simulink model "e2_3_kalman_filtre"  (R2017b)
settings: Solver=FixedStepAuto  StartTime=0.0  StopTime=30  FixedStep=fixed_step_size  RelTol=1e-3
StopFcn:
  | if AUTOLAND
  | %1_2
  | land1 = rospublisher('/tello1/land','std_msgs/Empty');
  | msg=rosmessage(land1);
  | send(land1,msg);
  | land2 = rospublisher('/tello2/land','std_msgs/Empty');
  | msg=rosmessage(land2);
  | send(land2,msg);
  | %3_4
  | land3 = rospublisher('/tello3/land','std_msgs/Empty');
  | msg=rosmessage(land3);
  | send(land3,msg);
  | land4 = rospublisher('/tello4/land','std_msgs/Empty');
  | msg=rosmessage(land4);
  | send(land4,msg);
  | %5_6
  | land5 = rospublisher('/tello5/land','std_msgs/Empty');
  | msg=rosmessage(land5);
  | send(land5,msg);
  | land6= rospublisher('/tello6/land','std_msgs/Empty');
  | msg=rosmessage(land6);
  | send(land6,msg);
  | %7_8
  | land7 = rospublisher('/tello7/land','std_msgs/Empty');
  | msg=rosmessage(land7);
  | send(land7,msg);
  | land8 = rospublisher('/tello8/land','std_msgs/Empty');
  | msg=rosmessage(land8);
  | send(land8,msg);
  | end
  | 
  | generate_cifer_datapack
  | 
  | if TELLO_PLOT
  | tello8_plot
  | end
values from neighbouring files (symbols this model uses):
  a = XMAX    (= 0.8)    [start_tello.m]
  b = YMAX    (= 1.2)    [start_tello.m]
  battery_threshold = 15    [start_tello.m]
  bb = (ZMIN*YMAX - ZMAX*YMIN)/(YMAX - YMIN)    (= -1.05)    [start_tello.m]
  fcnCmdMag = 1    [start.m]
  fcnNumber = 4    [start.m]
  fcnSinFreq = 50.0    (= 50)    [start.m]
  high_time = 5    [start.m]
  k = (ZMAX - ZMIN)/(YMAX - YMIN)    (= 0.458333333333)    [start_tello.m]
  omega = 1.0    (= 1)    [start.m]    (also in start_tello.m = 0.3)
  PARAM_C1 = 4.0    (= 4)    [start.m]
  PARAM_C2 = 0.0187    [start.m]
  PARAM_isNoiseOn = false    [start.m]
  PARAM_T_rec = ceil(5*2*pi/PARAM_w_min)    [start.m]
  PARAM_time_end = PARAM_time_start + 20    (= 23)    [start.m]
  PARAM_time_start = 3    [start.m]
  PARAM_w_max = 12    [start.m]
  PARAM_w_min = 0.5    [start.m]
  R = 1.0    (= 1)    [start.m]    (also in start_tello.m)
  sim_end_time = 15*act_end + 4    (= 475.238898038)    [start_tello.m]
  step_period = zero1_time+high_time+zero2_time+low_time    (= 18)    [start.m]
  tb2 = tb    (= 2.7)    [start_tello.m]
  tb3 = tb*2    (= 5.4)    [start_tello.m]
  tb4 = tb*3    (= 8.1)    [start_tello.m]
  tb5 = tb*4    (= 10.8)    [start_tello.m]
  tb6 = tb*5    (= 13.5)    [start_tello.m]
  tb7 = tb*6    (= 16.2)    [start_tello.m]
  tb8 = tb*7    (= 18.9)    [start_tello.m]
  TELLO1_NUM = uint8(1)    [start_tello.m]
  TELLO2_NUM = uint8(2)    [start_tello.m]
  TELLO3_NUM = uint8(3)    [start_tello.m]
  TELLO4_NUM = uint8(4)    [start_tello.m]
  TELLO5_NUM = uint8(5)    [start_tello.m]
  TELLO6_NUM = uint8(6)    [start_tello.m]
  TELLO7_NUM = uint8(7)    [start_tello.m]
  TELLO8_NUM = uint8(8)    [start_tello.m]
  UAV_NUM = 0    [start_tello.m]
  w1 = 0.4    [start_tello.m]
  w2 = 0.2    [start_tello.m]
  z_d_for_land = -0.2    [start_tello.m]
  zero1_time = 3    [start.m]
  zero2_time = 5    [start.m]
  zero3_time = 5    [start.m]
undefined symbols (not defined in the file or in its folder): DiscIntNeverNeededParam, sigbuilder_block
libraries: simulink x45, etargetslib x24, dspnetwork x24, sharedtransform x8, aerolibanimutils x1
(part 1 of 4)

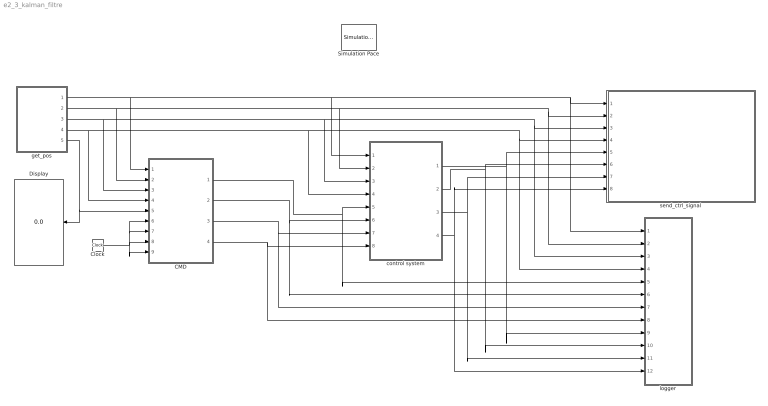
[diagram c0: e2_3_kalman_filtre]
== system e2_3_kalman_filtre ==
  CMD : Subsystem
  Clock : Clock
  Display : Display
  Simulation Pace : aerolibanimutils/Simulation Pace  SimulationPace=1  SleepMode=MATLAB Thread  OutputPaceError=off  SampleTime=-1
  control system : Subsystem
  get_pos : Subsystem
  logger : Subsystem  Commented=on
  send_ctrl_signal : Subsystem
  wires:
  control system/1(output1_2) -> logger/9(u1_2), send_ctrl_signal/5(control1_2)
  CMD/1(state_d1_2) -> logger/5(state_d1_2), control system/5(state_d1_2)
  CMD/2(state_d3_4) -> logger/6(state_d3_4), control system/6(state_d3_4)
  CMD/3(state_d5_6) -> logger/7(state_d5_6), control system/7(state_d5_6)
  CMD/4(state_d7_8) -> control system/8(state_d7_8), logger/8(state_d7_8)
  control system/2(output3_4) -> logger/10(u3_4), send_ctrl_signal/6(control3_4)
  control system/3(output5_6) -> logger/11(u5_6), send_ctrl_signal/7(control5_6)
  control system/4(output7_8) -> logger/12(u7_8), send_ctrl_signal/8(control7_8)
  get_pos/1(tello1_2) -> CMD/1(telo_state1_2), send_ctrl_signal/1(state1_2), logger/1(state1_2), control system/1(state1_2)
  get_pos/2(tello3_4) -> CMD/2(telo_state3_4), logger/2(state3_4), send_ctrl_signal/2(state3_4), control system/2(state3_4)
  get_pos/3(tello5_6) -> CMD/3(telo_state5_6), logger/3(state5_6), send_ctrl_signal/3(state5_6), control system/3(state5_6)
  get_pos/4(tello7_8) -> CMD/4(telo_state7_8), logger/4(state7_8), send_ctrl_signal/4(state7_8), control system/4(state7_8)
  Clock/1 -> CMD/6(clock1_2), CMD/7(clock3_4), CMD/8(clock5_6), CMD/9(clock7_8)
  get_pos/5(tello_bat) -> Display/1, CMD/5(tello_bat)

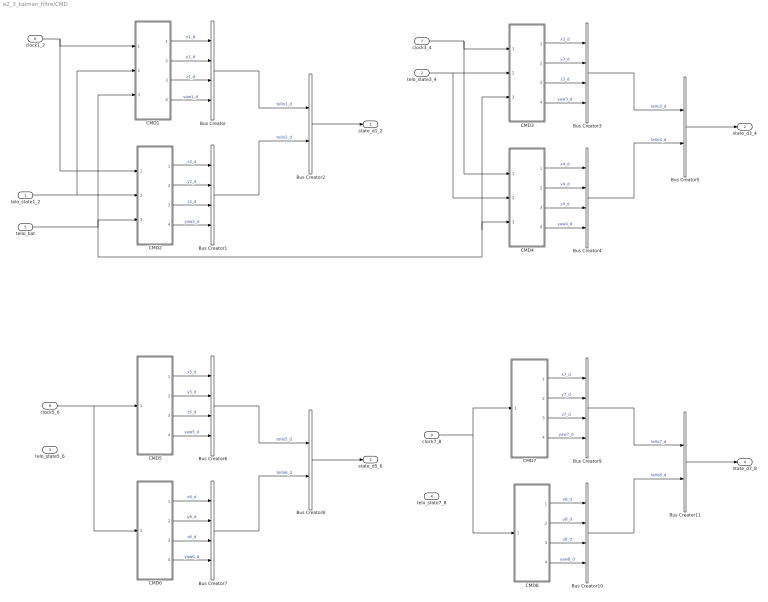
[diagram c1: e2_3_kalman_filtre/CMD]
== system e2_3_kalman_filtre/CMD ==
  telo_state1_2 : Inport
  telo_state3_4 : Inport  Port=2
  telo_state5_6 : Inport  Port=3
  telo_state7_8 : Inport  Port=4
  tello_bat : Inport  Port=5
  clock1_2 : Inport  Port=6
  clock3_4 : Inport  Port=7
  clock5_6 : Inport  Port=8
  clock7_8 : Inport  Port=9
  Bus Creator{,1,3..4,6..7,9..10} (8 alike) : BusCreator  Inputs=4
  Bus Creator{2,5,8,11} (4 alike) : BusCreator  Inputs=2
  CMD1 : Subsystem
  CMD2 : Subsystem
  CMD3 : Subsystem
  CMD4 : Subsystem
  CMD5 : Subsystem
  CMD6 : Subsystem
  CMD7 : Subsystem
  CMD8 : Subsystem
  state_d1_2 : Outport
  state_d3_4 : Outport  Port=2
  state_d5_6 : Outport  Port=3
  state_d7_8 : Outport  Port=4
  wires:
  CMD1/1(x_d) -> Bus Creator/1  "x1_d"
  CMD1/2(y_d) -> Bus Creator/2  "y1_d"
  CMD1/3(z_d) -> Bus Creator/3  "z1_d"
  CMD1/4(yaw_d) -> Bus Creator/4  "yaw1_d"
  CMD2/1(x_d) -> Bus Creator1/1  "x2_d"
  CMD2/2(y_d) -> Bus Creator1/2  "y2_d"
  CMD2/3(z_d) -> Bus Creator1/3  "z2_d"
  CMD2/4(yaw_d) -> Bus Creator1/4  "yaw2_d"
  Bus Creator/1 -> Bus Creator2/1  "tello1_d"
  Bus Creator1/1 -> Bus Creator2/2  "tello2_d"
  Bus Creator2/1 -> state_d1_2/1
  Bus Creator3/1 -> Bus Creator5/1  "tello3_d"
  Bus Creator4/1 -> Bus Creator5/2  "tello4_d"
  CMD3/2(y_d) -> Bus Creator3/2  "y3_d"
  CMD3/3(z_d) -> Bus Creator3/3  "z3_d"
  CMD3/4(yaw_d) -> Bus Creator3/4  "yaw3_d"
  Bus Creator5/1 -> state_d3_4/1
  CMD4/1(x_d) -> Bus Creator4/1  "x4_d"
  CMD3/1(x_d) -> Bus Creator3/1  "x3_d"
  CMD4/2(y_d) -> Bus Creator4/2  "y4_d"
  CMD4/4(yaw_d) -> Bus Creator4/4  "yaw4_d"
  CMD4/3(z_d) -> Bus Creator4/3  "z4_d"
  CMD5/2(y_d) -> Bus Creator6/2  "y5_d"
  Bus Creator11/1 -> state_d7_8/1
  CMD7/3(z_d) -> Bus Creator9/3  "z7_d"
  Bus Creator6/1 -> Bus Creator8/1  "tello5_d"
  CMD8/3(z_d) -> Bus Creator10/3  "z8_d"
  CMD8/4(yaw_d) -> Bus Creator10/4  "yaw8_d"
  CMD5/3(z_d) -> Bus Creator6/3  "z5_d"
  CMD7/4(yaw_d) -> Bus Creator9/4  "yaw7_d"
  CMD5/4(yaw_d) -> Bus Creator6/4  "yaw5_d"
  CMD7/2(y_d) -> Bus Creator9/2  "y7_d"
  Bus Creator7/1 -> Bus Creator8/2  "tello6_d"
  CMD8/1(x_d) -> Bus Creator10/1  "x8_d"
  Bus Creator9/1 -> Bus Creator11/1  "tello7_d"
  Bus Creator10/1 -> Bus Creator11/2  "tello8_d"
  clock1_2/1 -> CMD2/1("clock "), CMD1/1("clock ")
  CMD6/2(y_d) -> Bus Creator7/2  "y6_d"
  CMD6/4(yaw_d) -> Bus Creator7/4  "yaw6_d"
  CMD6/1(x_d) -> Bus Creator7/1  "x6_d"
  CMD7/1(x_d) -> Bus Creator9/1  "x7_d"
  CMD5/1(x_d) -> Bus Creator6/1  "x5_d"
  Bus Creator8/1 -> state_d5_6/1
  CMD8/2(y_d) -> Bus Creator10/2  "y8_d"
  CMD6/3(z_d) -> Bus Creator7/3  "z6_d"
  clock5_6/1 -> CMD6/1("clock "), CMD5/1("clock ")
  clock7_8/1 -> CMD7/1("clock "), CMD8/1("clock ")
  clock3_4/1 -> CMD4/1("clock "), CMD3/1("clock ")
  telo_state1_2/1 -> CMD1/2(tello_states), CMD2/2(tello_states)
  tello_bat/1 -> CMD1/3(tello_bat), CMD3/3(tello_bat), CMD4/3(tello_bat), CMD2/3(tello_bat)
  telo_state3_4/1 -> CMD4/2(tello_states), CMD3/2(tello_states)

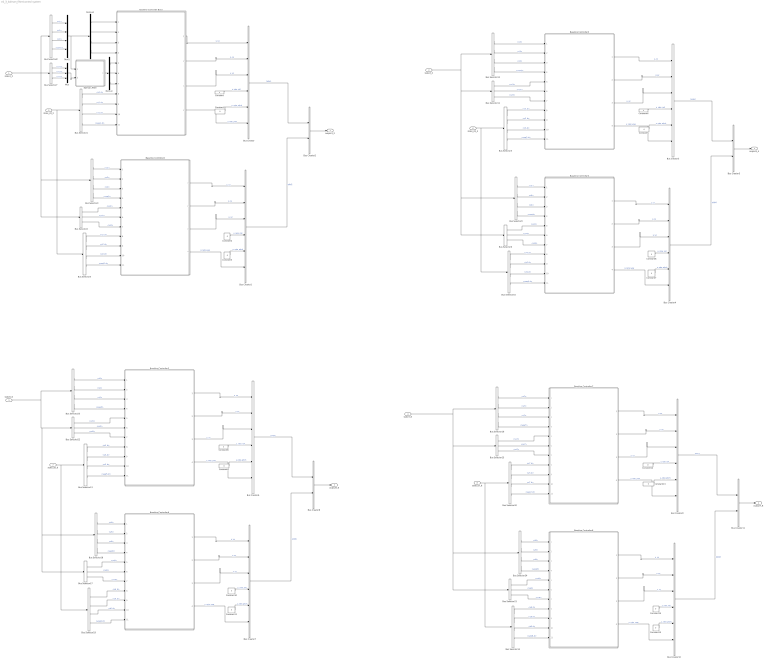
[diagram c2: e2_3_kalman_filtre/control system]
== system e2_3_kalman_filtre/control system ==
  state1_2 : Inport
  state3_4 : Inport  Port=2
  state5_6 : Inport  Port=3
  state7_8 : Inport  Port=4
  state_d1_2 : Inport  Port=5
  state_d3_4 : Inport  Port=6
  state_d5_6 : Inport  Port=7
  state_d7_8 : Inport  Port=8
  Baseline Controller Basic : Subsystem  AncestorBlock=ARBlocks/Baseline Controller
  Baseline Controller2 : Subsystem  AncestorBlock=ARBlocks/Baseline Controller
  Baseline Controller3 : Subsystem  AncestorBlock=ARBlocks/Baseline Controller
  Baseline Controller4 : Subsystem  AncestorBlock=ARBlocks/Baseline Controller
  Baseline Controller5 : Subsystem  AncestorBlock=ARBlocks/Baseline Controller
  Baseline Controller6 : Subsystem  AncestorBlock=ARBlocks/Baseline Controller
  Baseline Controller7 : Subsystem  AncestorBlock=ARBlocks/Baseline Controller
  Baseline Controller8 : Subsystem  AncestorBlock=ARBlocks/Baseline Controller
  Bus Creator{,1,3..4,6..7,9..10} (8 alike) : BusCreator  Inputs=6
  Bus Creator{2,5,8,11} (4 alike) : BusCreator  Inputs=2
  Bus Selector1 : BusSelector  OutputSignals=tello1_d.x1_d,tello1_d.y1_d,tello1_d.z1_d,tello1_d.yaw1_d
  Bus Selector10 : BusSelector  OutputSignals=tello4_d.x4_d,tello4_d.y4_d,tello4_d.z4_d,tello4_d.yaw4_d
  Bus Selector11 : BusSelector  OutputSignals=tello3_states.vx3,tello3_states.vy3,tello3_states.vz3
  Bus Selector12 : BusSelector  OutputSignals=tello3_states.x3,tello3_states.y3,tello3_states.z3,tello3_states.yaw3
  Bus Selector13 : BusSelector  OutputSignals=tello5_d.x5_d,tello5_d.y5_d,tello5_d.z5_d,tello5_d.yaw5_d
  Bus Selector14 : BusSelector  OutputSignals=tello8_d.x8_d,tello8_d.y8_d,tello8_d.z8_d,tello8_d.yaw8_d
  Bus Selector15 : BusSelector  OutputSignals=tello7_states.vx7,tello7_states.vy7,tello7_states.vz7
  Bus Selector16 : BusSelector  OutputSignals=tello7_states.x7,tello7_states.y7,tello7_states.z7,tello7_states.yaw7
  Bus Selector17 : BusSelector  OutputSignals=tello6_states.vx6,tello6_states.vy6,tello6_states.vz6
  Bus Selector18 : BusSelector  OutputSignals=tello6_states.x6,tello6_states.y6,tello6_states.z6,tello6_states.yaw6
  Bus Selector19 : BusSelector  OutputSignals=tello6_d.x6_d,tello6_d.y6_d,tello6_d.z6_d,tello6_d.yaw6_d
  Bus Selector2 : BusSelector  OutputSignals=tello2_states.vx2,tello2_states.vy2,tello2_states.vz2
  Bus Selector20 : BusSelector  OutputSignals=tello7_d.x7_d,tello7_d.y7_d,tello7_d.z7_d,tello7_d.yaw7_d
  Bus Selector21 : BusSelector  OutputSignals=tello8_states.vx8,tello8_states.vy8,tello8_states.vz8
  Bus Selector22 : BusSelector  OutputSignals=tello5_states.vx5,tello5_states.vy5,tello5_states.vz5
  Bus Selector23 : BusSelector  OutputSignals=tello5_states.x5,tello5_states.y5,tello5_states.z5,tello5_states.yaw5
  Bus Selector24 : BusSelector  OutputSignals=tello8_states.x8,tello8_states.y8,tello8_states.z8,tello8_states.yaw8
  Bus Selector3 : BusSelector  OutputSignals=tello2_states.x2,tello2_states.y2,tello2_states.z2,tello2_states.yaw2
  Bus Selector4 : BusSelector  OutputSignals=tello2_d.x2_d,tello2_d.y2_d,tello2_d.z2_d,tello2_d.yaw2_d
  Bus Selector5 : BusSelector  OutputSignals=tello3_d.x3_d,tello3_d.y3_d,tello3_d.z3_d,tello3_d.yaw3_d
  Bus Selector6 : BusSelector  OutputSignals=tello4_states.vx4,tello4_states.vy4,tello4_states.vz4
  Bus Selector7 : BusSelector  OutputSignals=tello1_states.vx1,tello1_states.vy1,tello1_states.vz1
  Bus Selector8 : BusSelector  OutputSignals=tello1_states.x1,tello1_states.y1,tello1_states.z1,tello1_states.yaw1
  Bus Selector9 : BusSelector  OutputSignals=tello4_states.x4,tello4_states.y4,tello4_states.z4,tello4_states.yaw4
  Constant{,1..15} (16 alike) : Constant  Value=0
  Demux : Demux  Outputs=3
  Demux1 : Demux
  Kalman_Filtre : Subsystem
  Mux : Mux  Inputs=3
  Mux1 : Mux
  output1_2 : Outport
  output3_4 : Outport  Port=2
  output5_6 : Outport  Port=3
  output7_8 : Outport  Port=4
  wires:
  Bus Selector1/2 -> Baseline Controller Basic/9(y_d)  "<y1_d>"
  Bus Selector8/3 -> Mux1/3  "<z1>"
  Bus Selector1/3 -> Baseline Controller Basic/10(Z_d)  "<z1_d>"
  Bus Selector8/4 -> Mux1/4  "<yaw1>"
  Bus Selector2/2 -> Baseline Controller2/6(V_y)  "<vy2>"
  Bus Selector3/4 -> Baseline Controller2/4(Yaw_e)  "<yaw2>"
  Bus Selector3/2 -> Baseline Controller2/2(Y_e)  "<y2>"
  Bus Selector1/1 -> Baseline Controller Basic/8(x_d)  "<x1_d>"
  Bus Selector7/1 -> Mux/1  "<vx1>"
  Bus Selector3/1 -> Baseline Controller2/1(X_e)  "<x2>"
  Bus Selector2/3 -> Baseline Controller2/7("V_z ")  "<vz2>"
  Bus Selector7/2 -> Mux/2  "<vy1>"
  Bus Selector2/1 -> Baseline Controller2/5(" V_x")  "<vx2>"
  Bus Selector8/1 -> Mux1/1  "<x1>"
  Bus Selector3/3 -> Baseline Controller2/3(" Z_e ")  "<z2>"
  Bus Selector1/4 -> Baseline Controller Basic/11(Yaw_d)  "<yaw1_d>"
  Bus Selector8/2 -> Mux1/2  "<y1>"
  Bus Selector7/3 -> Mux/3  "<vz1>"
  Baseline Controller Basic/1(ux) -> Bus Creator/1  "u_vx"
  Baseline Controller Basic/2(uy) -> Bus Creator/2  "u_vy"
  Baseline Controller Basic/3(Z_velocity_d. [-1,1]) -> Bus Creator/3  "u_vz"
  Baseline Controller Basic/4(yaw_rate_d [-1,1]) -> Bus Creator/6  "u_rate_yaw"
  Constant/1 -> Bus Creator/4  "u_rate_roll"
  Constant1/1 -> Bus Creator/5  "u_rate_pitch"
  Baseline Controller2/4(yaw_rate_d [-1,1]) -> Bus Creator1/6  "u_rate_yaw"
  Baseline Controller2/1(ux) -> Bus Creator1/1  "u_vx"
  Constant2/1 -> Bus Creator1/4  "u_rate_roll"
  Baseline Controller2/2(uy) -> Bus Creator1/2  "u_vy"
  Baseline Controller2/3(Z_velocity_d. [-1,1]) -> Bus Creator1/3  "u_vz"
  Constant3/1 -> Bus Creator1/5  "u_rate_pitch"
  Bus Creator/1 -> Bus Creator2/1  "tello1"
  Bus Creator1/1 -> Bus Creator2/2  "tello2"
  Bus Creator2/1 -> output1_2/1
  state_d1_2/1 -> Bus Selector4/1, Bus Selector1/1
  Bus Selector4/1 -> Baseline Controller2/8(x_d)  "<x2_d>"
  Bus Selector4/3 -> Baseline Controller2/10(Z_d)  "<z2_d>"
  Bus Selector4/2 -> Baseline Controller2/9(y_d)  "<y2_d>"
  Bus Selector4/4 -> Baseline Controller2/11(Yaw_d)  "<yaw2_d>"
  Bus Selector6/3 -> Baseline Controller4/7("V_z ")  "<vz4>"
  Bus Selector6/1 -> Baseline Controller4/5(" V_x")  "<vx4>"
  Bus Selector12/4 -> Baseline Controller3/4(Yaw_e)  "<yaw3>"
  Constant4/1 -> Bus Creator3/4  "u_rate_roll"
  Baseline Controller4/3(Z_velocity_d. [-1,1]) -> Bus Creator4/3  "u_vz"
  Baseline Controller3/3(Z_velocity_d. [-1,1]) -> Bus Creator3/3  "u_vz"
  Bus Selector5/4 -> Baseline Controller3/11(Yaw_d)  "<yaw3_d>"
  Baseline Controller4/1(ux) -> Bus Creator4/1  "u_vx"
  Bus Selector10/1 -> Baseline Controller4/8(x_d)  "<x4_d>"
  Bus Selector12/2 -> Baseline Controller3/2(Y_e)  "<y3>"
  Baseline Controller4/4(yaw_rate_d [-1,1]) -> Bus Creator4/6  "u_rate_yaw"
  Bus Selector5/3 -> Baseline Controller3/10(Z_d)  "<z3_d>"
  Bus Selector11/3 -> Baseline Controller3/7("V_z ")  "<vz3>"
  Bus Selector12/1 -> Baseline Controller3/1(X_e)  "<x3>"
  Bus Selector10/2 -> Baseline Controller4/9(y_d)  "<y4_d>"
  Bus Selector9/4 -> Baseline Controller4/4(Yaw_e)  "<yaw4>"
  Bus Selector12/3 -> Baseline Controller3/3(" Z_e ")  "<z3>"
  Baseline Controller4/2(uy) -> Bus Creator4/2  "u_vy"
  Constant7/1 -> Bus Creator4/5  "u_rate_pitch"
  Bus Selector6/2 -> Baseline Controller4/6(V_y)  "<vy4>"
  Baseline Controller3/1(ux) -> Bus Creator3/1  "u_vx"
  Bus Selector9/1 -> Baseline Controller4/1(X_e)  "<x4>"
  Bus Selector5/2 -> Baseline Controller3/9(y_d)  "<y3_d>"
  Bus Selector11/2 -> Baseline Controller3/6(V_y)  "<vy3>"
  state_d3_4/1 -> Bus Selector10/1, Bus Selector5/1
  Bus Selector10/4 -> Baseline Controller4/11(Yaw_d)  "<yaw4_d>"
  Constant5/1 -> Bus Creator3/5  "u_rate_pitch"
  Bus Selector11/1 -> Baseline Controller3/5(" V_x")  "<vx3>"
  Bus Selector5/1 -> Baseline Controller3/8(x_d)  "<x3_d>"
  Constant6/1 -> Bus Creator4/4  "u_rate_roll"
  Bus Creator5/1 -> output3_4/1
  Bus Selector10/3 -> Baseline Controller4/10(Z_d)  "<z4_d>"
  Bus Selector9/2 -> Baseline Controller4/2(Y_e)  "<y4>"
  Bus Creator3/1 -> Bus Creator5/1  "tello3"
  Bus Selector9/3 -> Baseline Controller4/3(" Z_e ")  "<z4>"
  Baseline Controller3/4(yaw_rate_d [-1,1]) -> Bus Creator3/6  "u_rate_yaw"
  Baseline Controller3/2(uy) -> Bus Creator3/2  "u_vy"
  Bus Creator4/1 -> Bus Creator5/2  "tello4"
  Bus Selector17/1 -> Baseline Controller6/5(" V_x")  "<vx6>"
  Bus Selector24/4 -> Baseline Controller8/4(Yaw_e)  "<yaw8>"
  Bus Selector16/3 -> Baseline Controller7/3(" Z_e ")  "<z7>"
  Baseline Controller8/4(yaw_rate_d [-1,1]) -> Bus Creator10/6  "u_rate_yaw"
  Bus Selector23/2 -> Baseline Controller5/2(Y_e)  "<y5>"
  Baseline Controller5/1(ux) -> Bus Creator6/1  "u_vx"
  Bus Selector16/1 -> Baseline Controller7/1(X_e)  "<x7>"
  Bus Selector13/4 -> Baseline Controller5/11(Yaw_d)  "<yaw5_d>"
  Bus Selector24/1 -> Baseline Controller8/1(X_e)  "<x8>"
  state_d5_6/1 -> Bus Selector19/1, Bus Selector13/1
  Bus Selector19/2 -> Baseline Controller6/9(y_d)  "<y6_d>"
  Constant12/1 -> Bus Creator9/4  "u_rate_roll"
  Constant15/1 -> Bus Creator10/5  "u_rate_pitch"
  Bus Creator9/1 -> Bus Creator11/1  "tello7"
  Bus Selector21/2 -> Baseline Controller8/6(V_y)  "<vy8>"
  Baseline Controller7/3(Z_velocity_d. [-1,1]) -> Bus Creator9/3  "u_vz"
  Baseline Controller6/3(Z_velocity_d. [-1,1]) -> Bus Creator7/3  "u_vz"
  Bus Selector14/4 -> Baseline Controller8/11(Yaw_d)  "<yaw8_d>"
  Bus Selector13/2 -> Baseline Controller5/9(y_d)  "<y5_d>"
  Baseline Controller8/2(uy) -> Bus Creator10/2  "u_vy"
  Baseline Controller6/2(uy) -> Bus Creator7/2  "u_vy"
  Bus Selector20/3 -> Baseline Controller7/10(Z_d)  "<z7_d>"
  Baseline Controller7/2(uy) -> Bus Creator9/2  "u_vy"
  Bus Selector18/1 -> Baseline Controller6/1(X_e)  "<x6>"
  Constant14/1 -> Bus Creator10/4  "u_rate_roll"
  Baseline Controller8/1(ux) -> Bus Creator10/1  "u_vx"
  Bus Selector19/1 -> Baseline Controller6/8(x_d)  "<x6_d>"
  Bus Selector22/2 -> Baseline Controller5/6(V_y)  "<vy5>"
  Bus Selector24/3 -> Baseline Controller8/3(" Z_e ")  "<z8>"
  Baseline Controller6/4(yaw_rate_d [-1,1]) -> Bus Creator7/6  "u_rate_yaw"
  Bus Selector16/2 -> Baseline Controller7/2(Y_e)  "<y7>"
  Bus Creator10/1 -> Bus Creator11/2  "tello8"
  Bus Selector23/1 -> Baseline Controller5/1(X_e)  "<x5>"
  Constant11/1 -> Bus Creator7/5  "u_rate_pitch"
  Constant8/1 -> Bus Creator6/4  "u_rate_roll"
  Baseline Controller6/1(ux) -> Bus Creator7/1  "u_vx"
  Bus Selector23/3 -> Baseline Controller5/3(" Z_e ")  "<z5>"
  Bus Selector13/3 -> Baseline Controller5/10(Z_d)  "<z5_d>"
  Bus Selector23/4 -> Baseline Controller5/4(Yaw_e)  "<yaw5>"
  Bus Selector22/3 -> Baseline Controller5/7("V_z ")  "<vz5>"
  Bus Selector19/4 -> Baseline Controller6/11(Yaw_d)  "<yaw6_d>"
  Bus Creator11/1 -> output7_8/1
  Bus Selector14/1 -> Baseline Controller8/8(x_d)  "<x8_d>"
  Baseline Controller8/3(Z_velocity_d. [-1,1]) -> Bus Creator10/3  "u_vz"
  state_d7_8/1 -> Bus Selector14/1, Bus Selector20/1
  Bus Selector21/1 -> Baseline Controller8/5(" V_x")  "<vx8>"
  Bus Selector16/4 -> Baseline Controller7/4(Yaw_e)  "<yaw7>"
  Bus Selector18/4 -> Baseline Controller6/4(Yaw_e)  "<yaw6>"
  Bus Selector17/3 -> Baseline Controller6/7("V_z ")  "<vz6>"
  Baseline Controller7/1(ux) -> Bus Creator9/1  "u_vx"
  Bus Selector14/3 -> Baseline Controller8/10(Z_d)  "<z8_d>"
  Constant13/1 -> Bus Creator9/5  "u_rate_pitch"
  Bus Selector15/1 -> Baseline Controller7/5(" V_x")  "<vx7>"
  Bus Selector14/2 -> Baseline Controller8/9(y_d)  "<y8_d>"
  Bus Selector22/1 -> Baseline Controller5/5(" V_x")  "<vx5>"
  Bus Selector15/3 -> Baseline Controller7/7("V_z ")  "<vz7>"
  Constant10/1 -> Bus Creator7/4  "u_rate_roll"
  Bus Selector21/3 -> Baseline Controller8/7("V_z ")  "<vz8>"
  Bus Selector15/2 -> Baseline Controller7/6(V_y)  "<vy7>"
  Bus Creator8/1 -> output5_6/1
  Baseline Controller5/3(Z_velocity_d. [-1,1]) -> Bus Creator6/3  "u_vz"
  state1_2/1 -> Bus Selector2/1, Bus Selector3/1, Bus Selector8/1, Bus Selector7/1
  Bus Creator7/1 -> Bus Creator8/2  "tello6"
  Bus Selector18/2 -> Baseline Controller6/2(Y_e)  "<y6>"
  Bus Creator6/1 -> Bus Creator8/1  "tello5"
  Bus Selector20/1 -> Baseline Controller7/8(x_d)  "<x7_d>"
  Bus Selector20/2 -> Baseline Controller7/9(y_d)  "<y7_d>"
  Baseline Controller7/4(yaw_rate_d [-1,1]) -> Bus Creator9/6  "u_rate_yaw"
  Bus Selector18/3 -> Baseline Controller6/3(" Z_e ")  "<z6>"
  Bus Selector24/2 -> Baseline Controller8/2(Y_e)  "<y8>"
  Constant9/1 -> Bus Creator6/5  "u_rate_pitch"
  Bus Selector20/4 -> Baseline Controller7/11(Yaw_d)  "<yaw7_d>"
  Bus Selector13/1 -> Baseline Controller5/8(x_d)  "<x5_d>"
  Bus Selector17/2 -> Baseline Controller6/6(V_y)  "<vy6>"
  Bus Selector19/3 -> Baseline Controller6/10(Z_d)  "<z6_d>"
  Baseline Controller5/4(yaw_rate_d [-1,1]) -> Bus Creator6/6  "u_rate_yaw"
  Baseline Controller5/2(uy) -> Bus Creator6/2  "u_vy"
  state3_4/1 -> Bus Selector12/1, Bus Selector6/1, Bus Selector9/1, Bus Selector11/1
  state5_6/1 -> Bus Selector23/1, Bus Selector17/1, Bus Selector18/1, Bus Selector22/1
  state7_8/1 -> Bus Selector16/1, Bus Selector21/1, Bus Selector24/1, Bus Selector15/1
  Mux/1 -> Kalman_Filtre/2(Velocity_Real)
  Kalman_Filtre/1(Velocity_Feedback) -> Demux/1
  Demux/2 -> Baseline Controller Basic/6(V_y)
  Demux/1 -> Baseline Controller Basic/5(" V_x")
  Demux/3 -> Baseline Controller Basic/7(V_z)
  Mux1/1 -> Kalman_Filtre/1(Pos_Real), Demux1/1
  Demux1/1 -> Baseline Controller Basic/1(X_e)
  Demux1/2 -> Baseline Controller Basic/2(Y_e)
  Demux1/3 -> Baseline Controller Basic/3(" Z_e ")
  Demux1/4 -> Baseline Controller Basic/4(Yaw_e)

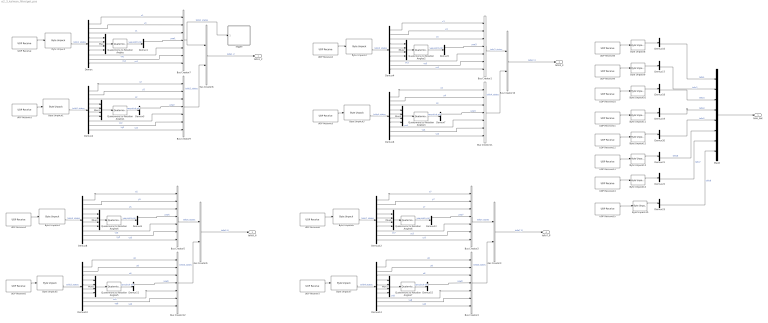
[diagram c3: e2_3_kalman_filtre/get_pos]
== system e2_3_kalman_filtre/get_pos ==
  Bus Creator{1..2,4..5,7,9,11..12} (8 alike) : BusCreator  Inputs=7
  Bus Creator{3,6,8,10} (4 alike) : BusCreator  Inputs=2
  Byte Unpack{,1..7} (8 alike) : etargetslib/Byte Unpack  dimensions={[1],10}  datatypes={'uint8','double'}  byteAlign=1
  Byte Unpack{8..15} (8 alike) : etargetslib/Byte Unpack  dimensions={[2],1}  datatypes={'uint8','double'}  byteAlign=1
  Demux{,2,4,6,8,10,12,14} (8 alike) : Demux  Outputs=10
  Demux{1,3,5,7,9,11,13,15} (8 alike) : Demux  Outputs=3
  Demux{16..23} (8 alike) : Demux  Outputs=2
  Mux{,1..7} (8 alike) : Mux
  Mux8 : Mux  Inputs=8
  Quaternions to Rotation Angles{,1..7} (8 alike) : sharedtransform/Quaternions to Rotation Angles  rotationOrder=ZYX
  UDP Receive : dspnetwork/UDP Receive  localURL='0.0.0.0'  localPort=TELLO1_REC_PORT  remoteURL=UDP_REC_IP  remotePort=-1  recvBufferSize=8192  dims=81  signalDatatype=uint8  isVarSize=off  showBlockingTime=off  blockingTime=0  sampletime=-1  blockPlatform=[]
  UDP Receive1 : dspnetwork/UDP Receive  localURL='0.0.0.0'  localPort=TELLO2_REC_PORT  remoteURL=UDP_REC_IP  remotePort=-1  recvBufferSize=8192  dims=81  signalDatatype=uint8  isVarSize=off  showBlockingTime=off  blockingTime=0  sampletime=-1  blockPlatform=[]
  UDP Receive10 : dspnetwork/UDP Receive  localURL='0.0.0.0'  localPort=26052  remoteURL='127.0.0.1'  remotePort=-1  recvBufferSize=100  dims=10  signalDatatype=uint8  isVarSize=off  showBlockingTime=off  blockingTime=0  sampletime=-1  blockPlatform=[]
  UDP Receive11 : dspnetwork/UDP Receive  localURL='0.0.0.0'  localPort=26053  remoteURL='127.0.0.1'  remotePort=-1  recvBufferSize=100  dims=10  signalDatatype=uint8  isVarSize=off  showBlockingTime=off  blockingTime=0  sampletime=-1  blockPlatform=[]
  UDP Receive12 : dspnetwork/UDP Receive  localURL='0.0.0.0'  localPort=26054  remoteURL='127.0.0.1'  remotePort=-1  recvBufferSize=100  dims=10  signalDatatype=uint8  isVarSize=off  showBlockingTime=off  blockingTime=0  sampletime=-1  blockPlatform=[]
  UDP Receive13 : dspnetwork/UDP Receive  localURL='0.0.0.0'  localPort=26055  remoteURL='127.0.0.1'  remotePort=-1  recvBufferSize=100  dims=10  signalDatatype=uint8  isVarSize=off  showBlockingTime=off  blockingTime=0  sampletime=-1  blockPlatform=[]
  UDP Receive14 : dspnetwork/UDP Receive  localURL='0.0.0.0'  localPort=26056  remoteURL='127.0.0.1'  remotePort=-1  recvBufferSize=100  dims=10  signalDatatype=uint8  isVarSize=off  showBlockingTime=off  blockingTime=0  sampletime=-1  blockPlatform=[]
  UDP Receive15 : dspnetwork/UDP Receive  localURL='0.0.0.0'  localPort=26057  remoteURL='127.0.0.1'  remotePort=-1  recvBufferSize=100  dims=10  signalDatatype=uint8  isVarSize=off  showBlockingTime=off  blockingTime=0  sampletime=-1  blockPlatform=[]
  UDP Receive2 : dspnetwork/UDP Receive  localURL='0.0.0.0'  localPort=TELLO3_REC_PORT  remoteURL=UDP_REC_IP  remotePort=-1  recvBufferSize=8192  dims=81  signalDatatype=uint8  isVarSize=off  showBlockingTime=off  blockingTime=0  sampletime=-1  blockPlatform=[]
  UDP Receive3 : dspnetwork/UDP Receive  localURL='0.0.0.0'  localPort=TELLO4_REC_PORT  remoteURL=UDP_REC_IP  remotePort=-1  recvBufferSize=8192  dims=81  signalDatatype=uint8  isVarSize=off  showBlockingTime=off  blockingTime=0  sampletime=-1  blockPlatform=[]
  UDP Receive4 : dspnetwork/UDP Receive  localURL='0.0.0.0'  localPort=TELLO5_REC_PORT  remoteURL=UDP_REC_IP  remotePort=-1  recvBufferSize=8192  dims=81  signalDatatype=uint8  isVarSize=off  showBlockingTime=off  blockingTime=0  sampletime=-1  blockPlatform=[]
  UDP Receive5 : dspnetwork/UDP Receive  localURL='0.0.0.0'  localPort=TELLO6_REC_PORT  remoteURL=UDP_REC_IP  remotePort=-1  recvBufferSize=8192  dims=81  signalDatatype=uint8  isVarSize=off  showBlockingTime=off  blockingTime=0  sampletime=-1  blockPlatform=[]
  UDP Receive6 : dspnetwork/UDP Receive  localURL='0.0.0.0'  localPort=TELLO7_REC_PORT  remoteURL=UDP_REC_IP  remotePort=-1  recvBufferSize=8192  dims=81  signalDatatype=uint8  isVarSize=off  showBlockingTime=off  blockingTime=0  sampletime=-1  blockPlatform=[]
  UDP Receive7 : dspnetwork/UDP Receive  localURL='0.0.0.0'  localPort=TELLO8_REC_PORT  remoteURL=UDP_REC_IP  remotePort=-1  recvBufferSize=8192  dims=81  signalDatatype=uint8  isVarSize=off  showBlockingTime=off  blockingTime=0  sampletime=-1  blockPlatform=[]
  UDP Receive8 : dspnetwork/UDP Receive  localURL='0.0.0.0'  localPort=26050  remoteURL='127.0.0.1'  remotePort=-1  recvBufferSize=100  dims=10  signalDatatype=uint8  isVarSize=off  showBlockingTime=off  blockingTime=0  sampletime=-1  blockPlatform=[]
  UDP Receive9 : dspnetwork/UDP Receive  localURL='0.0.0.0'  localPort=26051  remoteURL='127.0.0.1'  remotePort=-1  recvBufferSize=100  dims=10  signalDatatype=uint8  isVarSize=off  showBlockingTime=off  blockingTime=0  sampletime=-1  blockPlatform=[]
  logger : Subsystem
  tello1_2 : Outport
  tello3_4 : Outport  Port=2
  tello5_6 : Outport  Port=3
  tello7_8 : Outport  Port=4
  tello_bat : Outport  Port=5
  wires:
  Demux1/1 -> Bus Creator7/4  "yaw1"
  Byte Unpack/2 -> Demux/1  "tello1_states"
  Demux/2 -> Bus Creator7/2  "y1"
  Demux2/8 -> Bus Creator9/5  "vx2"
  Demux3/1 -> Bus Creator9/4  "yaw2"
  Demux/8 -> Bus Creator7/5  "vx1"
  Demux2/4 -> Mux1/1
  UDP Receive1/1 -> Byte Unpack1/1
  Demux/6 -> Mux/3
  Demux2/1 -> Bus Creator9/1  "x2"
  UDP Receive/1 -> Byte Unpack/1
  Demux2/3 -> Bus Creator9/3  "z2"
  Demux2/5 -> Mux1/2
  Demux/10 -> Bus Creator7/7  "vz1"
  Demux/4 -> Mux/1
  Bus Creator8/1 -> tello1_2/1  "tello1_2"
  Demux2/7 -> Mux1/4
  Demux/1 -> Bus Creator7/1  "x1"
  Demux2/10 -> Bus Creator9/7  "vz2"
  Demux2/6 -> Mux1/3
  Demux2/9 -> Bus Creator9/6  "vy2"
  Quaternions to Rotation Angles1/1 -> Demux3/1  "yaw-pitch-roll"
  Bus Creator9/1 -> Bus Creator8/2  "tello2_states"
  Mux1/1 -> Quaternions to Rotation Angles1/1
  Demux/3 -> Bus Creator7/3  "z1"
  Demux/7 -> Mux/4
  Quaternions to Rotation Angles/1 -> Demux1/1  "yaw-pitch-roll"
  Demux/9 -> Bus Creator7/6  "vy1"
  Demux/5 -> Mux/2
  Byte Unpack1/2 -> Demux2/1  "tello2_states"
  Mux/1 -> Quaternions to Rotation Angles/1
  Demux2/2 -> Bus Creator9/2  "y2"
  Demux6/9 -> Bus Creator11/6  "vy4"
  Demux6/6 -> Mux3/3
  Demux6/10 -> Bus Creator11/7  "vz4"
  Demux4/1 -> Bus Creator1/1  "x3"
  Demux4/4 -> Mux2/1
  Demux4/9 -> Bus Creator1/6  "vy3"
  Demux4/10 -> Bus Creator1/7  "vz3"
  Demux5/1 -> Bus Creator1/4  "yaw3"
  UDP Receive2/1 -> Byte Unpack2/1
  Demux4/6 -> Mux2/3
  UDP Receive3/1 -> Byte Unpack3/1
  Demux6/7 -> Mux3/4
  Demux4/2 -> Bus Creator1/2  "y3"
  Bus Creator1/1 -> Bus Creator10/1  "tello3_states"
  Demux4/8 -> Bus Creator1/5  "vx3"
  Byte Unpack3/2 -> Demux6/1  "tello4_states"
  Demux6/1 -> Bus Creator11/1  "x4"
  Byte Unpack2/2 -> Demux4/1  "tello3_states"
  Demux6/3 -> Bus Creator11/3  "z4"
  Demux6/8 -> Bus Creator11/5  "vx4"
  Quaternions to Rotation Angles3/1 -> Demux7/1  "yaw-pitch-roll"
  Demux7/1 -> Bus Creator11/4  "yaw4"
  Bus Creator10/1 -> tello3_4/1  "tello3_4"
  Demux6/5 -> Mux3/2
  Demux6/4 -> Mux3/1
  Bus Creator11/1 -> Bus Creator10/2  "tello4_states"
  Mux3/1 -> Quaternions to Rotation Angles3/1
  Demux4/3 -> Bus Creator1/3  "z3"
  Demux4/7 -> Mux2/4
  Quaternions to Rotation Angles2/1 -> Demux5/1  "yaw-pitch-roll"
  Demux4/5 -> Mux2/2
  Mux2/1 -> Quaternions to Rotation Angles2/1
  Demux6/2 -> Bus Creator11/2  "y4"
  Demux10/6 -> Mux5/3
  Demux10/10 -> Bus Creator12/7  "vz6"
  Demux8/10 -> Bus Creator5/7  "vz5"
  Demux8/1 -> Bus Creator5/1  "x5"
  Demux10/5 -> Mux5/2
  UDP Receive4/1 -> Byte Unpack4/1
  Demux14/4 -> Mux7/1
  Demux10/1 -> Bus Creator12/1  "x6"
  Demux8/6 -> Mux4/3
  Bus Creator12/1 -> Bus Creator6/2  "tello6_states"
  UDP Receive5/1 -> Byte Unpack5/1
  Demux10/8 -> Bus Creator12/5  "vx6"
  Demux14/10 -> Bus Creator4/7  "vz8"
  Demux10/4 -> Mux5/1
  Demux9/1 -> Bus Creator5/4  "yaw5"
  Demux8/8 -> Bus Creator5/5  "vx5"
  Bus Creator5/1 -> Bus Creator6/1  "tello5_states"
  Demux10/3 -> Bus Creator12/3  "z6"
  Demux8/2 -> Bus Creator5/2  "y5"
  Demux12/2 -> Bus Creator2/2  "y7"
  Demux14/3 -> Bus Creator4/3  "z8"
  Mux7/1 -> Quaternions to Rotation Angles7/1
  Bus Creator4/1 -> Bus Creator3/2  "tello8_states"
  Demux14/9 -> Bus Creator4/6  "vy8"
  Demux12/5 -> Mux6/2
  Demux8/5 -> Mux4/2
  Demux12/9 -> Bus Creator2/6  "vy7"
  Demux14/5 -> Mux7/2
  UDP Receive7/1 -> Byte Unpack7/1
  Demux12/1 -> Bus Creator2/1  "x7"
  Demux14/8 -> Bus Creator4/5  "vx8"
  Quaternions to Rotation Angles7/1 -> Demux15/1  "yaw-pitch-roll"
  Demux12/10 -> Bus Creator2/7  "vz7"
  Demux14/1 -> Bus Creator4/1  "x8"
  Bus Creator6/1 -> tello5_6/1  "tello5_6"
  Demux8/7 -> Mux4/4
  Bus Creator2/1 -> Bus Creator3/1  "tello7_states"
  Demux10/7 -> Mux5/4
  Mux5/1 -> Quaternions to Rotation Angles5/1
  Demux11/1 -> Bus Creator12/4  "yaw6"
  Demux13/1 -> Bus Creator2/4  "yaw7"
  Demux14/7 -> Mux7/4
  Demux15/1 -> Bus Creator4/4  "yaw8"
  Demux12/3 -> Bus Creator2/3  "z7"
  Byte Unpack4/2 -> Demux8/1  "tello5_states"
  Demux10/2 -> Bus Creator12/2  "y6"
  Demux14/2 -> Bus Creator4/2  "y8"
  Bus Creator3/1 -> tello7_8/1  "tello7_8"
  Byte Unpack6/2 -> Demux12/1  "tello7_states"
  Demux12/7 -> Mux6/4
  Demux12/4 -> Mux6/1
  Demux8/4 -> Mux4/1
  Quaternions to Rotation Angles6/1 -> Demux13/1  "yaw-pitch-roll"
  Mux6/1 -> Quaternions to Rotation Angles6/1
  Demux10/9 -> Bus Creator12/6  "vy6"
  UDP Receive6/1 -> Byte Unpack6/1
  Demux12/6 -> Mux6/3
  Demux12/8 -> Bus Creator2/5  "vx7"
  Byte Unpack7/2 -> Demux14/1  "tello4_states"
  Quaternions to Rotation Angles5/1 -> Demux11/1  "yaw-pitch-roll"
  Demux8/3 -> Bus Creator5/3  "z5"
  Quaternions to Rotation Angles4/1 -> Demux9/1  "yaw-pitch-roll"
  Demux8/9 -> Bus Creator5/6  "vy5"
  Byte Unpack5/2 -> Demux10/1  "tello2_states"
  Mux4/1 -> Quaternions to Rotation Angles4/1
  Demux14/6 -> Mux7/3
  UDP Receive8/1 -> Byte Unpack8/1
  UDP Receive9/1 -> Byte Unpack9/1
  UDP Receive10/1 -> Byte Unpack10/1
  UDP Receive11/1 -> Byte Unpack11/1
  UDP Receive12/1 -> Byte Unpack12/1
  UDP Receive13/1 -> Byte Unpack13/1
  UDP Receive14/1 -> Byte Unpack14/1
  UDP Receive15/1 -> Byte Unpack15/1
  Byte Unpack8/1 -> Demux16/1
  Demux16/2 -> Mux8/1  "tello1"
  Mux8/1 -> tello_bat/1
  Byte Unpack9/1 -> Demux17/1
  Byte Unpack10/1 -> Demux18/1
  Byte Unpack11/1 -> Demux19/1
  Byte Unpack12/1 -> Demux20/1
  Byte Unpack13/1 -> Demux21/1
  Byte Unpack14/1 -> Demux22/1
  Byte Unpack15/1 -> Demux23/1
  Demux17/2 -> Mux8/2  "tello2"
  Demux18/2 -> Mux8/3  "tello3"
  Demux19/2 -> Mux8/4  "tello4"
  Demux20/2 -> Mux8/5  "tello5"
  Demux21/2 -> Mux8/6  "tello6"
  Demux22/2 -> Mux8/7  "tello7"
  Demux23/2 -> Mux8/8  "tello8"
  Bus Creator7/1 -> logger/1(tello1_states), Bus Creator8/1  "tello1_states"

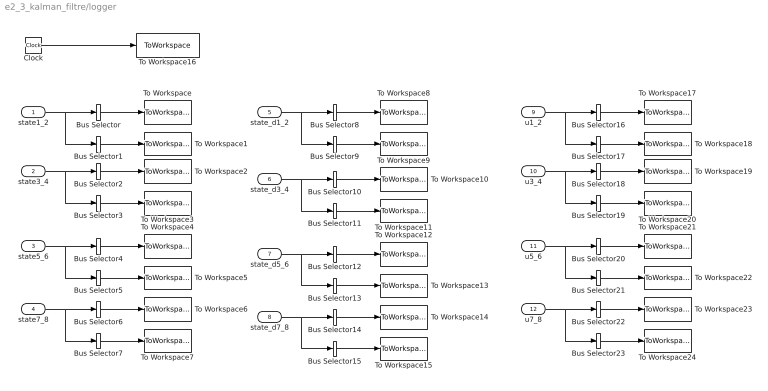
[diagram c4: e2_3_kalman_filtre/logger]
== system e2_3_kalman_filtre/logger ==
  state1_2 : Inport
  state3_4 : Inport  Port=2
  state5_6 : Inport  Port=3
  state7_8 : Inport  Port=4
  state_d1_2 : Inport  Port=5
  state_d3_4 : Inport  Port=6
  state_d5_6 : Inport  Port=7
  state_d7_8 : Inport  Port=8
  u1_2 : Inport  Port=9
  u3_4 : Inport  Port=10
  u5_6 : Inport  Port=11
  u7_8 : Inport  Port=12
  Bus Selector : BusSelector  OutputSignals=tello1_states.x1,tello1_states.y1,tello1_states.z1,tello1_states.yaw1,tello1_states.vx1,tello1_states.vy1,tello1_states.vz1  OutputAsBus=on
  Bus Selector1 : BusSelector  OutputSignals=tello2_states.x2,tello2_states.y2,tello2_states.z2,tello2_states.yaw2,tello2_states.vx2,tello2_states.vy2,tello2_states.vz2  OutputAsBus=on
  Bus Selector10 : BusSelector  OutputSignals=tello3_d.x3_d,tello3_d.y3_d,tello3_d.z3_d,tello3_d.yaw3_d  OutputAsBus=on
  Bus Selector11 : BusSelector  OutputSignals=tello4_d.x4_d,tello4_d.y4_d,tello4_d.z4_d,tello4_d.yaw4_d  OutputAsBus=on
  Bus Selector12 : BusSelector  OutputSignals=tello5_d.x5_d,tello5_d.y5_d,tello5_d.z5_d,tello5_d.yaw5_d  OutputAsBus=on
  Bus Selector13 : BusSelector  OutputSignals=tello6_d.x6_d,tello6_d.y6_d,tello6_d.z6_d,tello6_d.yaw6_d  OutputAsBus=on
  Bus Selector14 : BusSelector  OutputSignals=tello7_d.x7_d,tello7_d.y7_d,tello7_d.z7_d,tello7_d.yaw7_d  OutputAsBus=on
  Bus Selector15 : BusSelector  OutputSignals=tello8_d.x8_d,tello8_d.y8_d,tello8_d.z8_d,tello8_d.yaw8_d  OutputAsBus=on
  Bus Selector16 : BusSelector  OutputSignals=tello1.u_vx,tello1.u_vy,tello1.u_vz,tello1.u_rate_roll,tello1.u_rate_pitch,tello1.u_rate_yaw  OutputAsBus=on
  Bus Selector17 : BusSelector  OutputSignals=tello2.u_vx,tello2.u_vy,tello2.u_vz,tello2.u_rate_roll,tello2.u_rate_pitch,tello2.u_rate_yaw  OutputAsBus=on
  Bus Selector18 : BusSelector  OutputSignals=tello3.u_vx,tello3.u_vy,tello3.u_vz,tello3.u_rate_roll,tello3.u_rate_pitch,tello3.u_rate_yaw  OutputAsBus=on
  Bus Selector19 : BusSelector  OutputSignals=tello4.u_vx,tello4.u_vy,tello4.u_vz,tello4.u_rate_roll,tello4.u_rate_pitch,tello4.u_rate_yaw  OutputAsBus=on
  Bus Selector2 : BusSelector  OutputSignals=tello3_states.x3,tello3_states.y3,tello3_states.z3,tello3_states.yaw3,tello3_states.vx3,tello3_states.vy3,tello3_states.vz3  OutputAsBus=on
  Bus Selector20 : BusSelector  OutputSignals=tello5.u_vx,tello5.u_vy,tello5.u_vz,tello5.u_rate_roll,tello5.u_rate_pitch,tello5.u_rate_yaw  OutputAsBus=on
  Bus Selector21 : BusSelector  OutputSignals=tello6.u_vx,tello6.u_vy,tello6.u_vz,tello6.u_rate_roll,tello6.u_rate_pitch,tello6.u_rate_yaw  OutputAsBus=on
  Bus Selector22 : BusSelector  OutputSignals=tello7.u_vx,tello7.u_vy,tello7.u_vz,tello7.u_rate_roll,tello7.u_rate_pitch,tello7.u_rate_yaw  OutputAsBus=on
  Bus Selector23 : BusSelector  OutputSignals=tello8.u_vx,tello8.u_vy,tello8.u_vz,tello8.u_rate_roll,tello8.u_rate_pitch,tello8.u_rate_yaw  OutputAsBus=on
  Bus Selector3 : BusSelector  OutputSignals=tello4_states.x4,tello4_states.y4,tello4_states.z4,tello4_states.yaw4,tello4_states.vx4,tello4_states.vy4,tello4_states.vz4  OutputAsBus=on
  Bus Selector4 : BusSelector  OutputSignals=tello5_states.x5,tello5_states.y5,tello5_states.z5,tello5_states.yaw5,tello5_states.vx5,tello5_states.vy5,tello5_states.vz5  OutputAsBus=on
  Bus Selector5 : BusSelector  OutputSignals=tello6_states.x6,tello6_states.y6,tello6_states.z6,tello6_states.yaw6,tello6_states.vx6,tello6_states.vy6,tello6_states.vz6  OutputAsBus=on
  Bus Selector6 : BusSelector  OutputSignals=tello7_states.x7,tello7_states.y7,tello7_states.z7,tello7_states.yaw7,tello7_states.vx7,tello7_states.vy7,tello7_states.vz7  OutputAsBus=on
  Bus Selector7 : BusSelector  OutputSignals=tello8_states.x8,tello8_states.y8,tello8_states.z8,tello8_states.yaw8,tello8_states.vx8,tello8_states.vy8,tello8_states.vz8  OutputAsBus=on
  Bus Selector8 : BusSelector  OutputSignals=tello1_d.x1_d,tello1_d.y1_d,tello1_d.z1_d,tello1_d.yaw1_d  OutputAsBus=on
  Bus Selector9 : BusSelector  OutputSignals=tello2_d.x2_d,tello2_d.y2_d,tello2_d.z2_d,tello2_d.yaw2_d  OutputAsBus=on
  Clock : Clock
  To Workspace : ToWorkspace  VariableName=tello1_states  SampleTime=-1
  To Workspace1 : ToWorkspace  VariableName=tello2_states  SampleTime=-1
  To Workspace10 : ToWorkspace  VariableName=tello3_states_d  SampleTime=-1
  To Workspace11 : ToWorkspace  VariableName=tello4_states_d  SampleTime=-1
  To Workspace12 : ToWorkspace  VariableName=tello5_states_d  SampleTime=-1
  To Workspace13 : ToWorkspace  VariableName=tello6_states_d  SampleTime=-1
  To Workspace14 : ToWorkspace  VariableName=tello7_states_d  SampleTime=-1
  To Workspace15 : ToWorkspace  VariableName=tello8_states_d  SampleTime=-1
  To Workspace16 : ToWorkspace  VariableName=tello_timestamp  SampleTime=-1
  To Workspace17 : ToWorkspace  VariableName=tello1_u  SampleTime=-1
  To Workspace18 : ToWorkspace  VariableName=tello2_u  SampleTime=-1
  To Workspace19 : ToWorkspace  VariableName=tello3_u  SampleTime=-1
  To Workspace2 : ToWorkspace  VariableName=tello3_states  SampleTime=-1
  To Workspace20 : ToWorkspace  VariableName=tello4_u  SampleTime=-1
  To Workspace21 : ToWorkspace  VariableName=tello5_u  SampleTime=-1
  To Workspace22 : ToWorkspace  VariableName=tello6_u  SampleTime=-1
  To Workspace23 : ToWorkspace  VariableName=tello7_u  SampleTime=-1
  To Workspace24 : ToWorkspace  VariableName=tello8_u  SampleTime=-1
  To Workspace3 : ToWorkspace  VariableName=tello4_states  SampleTime=-1
  To Workspace4 : ToWorkspace  VariableName=tello5_states  SampleTime=-1
  To Workspace5 : ToWorkspace  VariableName=tello6_states  SampleTime=-1
  To Workspace6 : ToWorkspace  VariableName=tello7_states  SampleTime=-1
  To Workspace7 : ToWorkspace  VariableName=tello8_states  SampleTime=-1
  To Workspace8 : ToWorkspace  VariableName=tello1_states_d  SampleTime=-1
  To Workspace9 : ToWorkspace  VariableName=tello2_states_d  SampleTime=-1
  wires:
  state1_2/1 -> Bus Selector1/1, Bus Selector/1
  Bus Selector/1 -> To Workspace/1
  Bus Selector1/1 -> To Workspace1/1
  Bus Selector3/1 -> To Workspace3/1
  Bus Selector2/1 -> To Workspace2/1
  state3_4/1 -> Bus Selector3/1, Bus Selector2/1
  Bus Selector5/1 -> To Workspace5/1
  Bus Selector4/1 -> To Workspace4/1
  state5_6/1 -> Bus Selector5/1, Bus Selector4/1
  Bus Selector7/1 -> To Workspace7/1
  Bus Selector6/1 -> To Workspace6/1
  state7_8/1 -> Bus Selector7/1, Bus Selector6/1
  Bus Selector9/1 -> To Workspace9/1
  Bus Selector8/1 -> To Workspace8/1
  state_d1_2/1 -> Bus Selector9/1, Bus Selector8/1
  Bus Selector10/1 -> To Workspace10/1
  Bus Selector11/1 -> To Workspace11/1
  Bus Selector12/1 -> To Workspace12/1
  state_d3_4/1 -> Bus Selector11/1, Bus Selector10/1
  state_d5_6/1 -> Bus Selector13/1, Bus Selector12/1
  Bus Selector15/1 -> To Workspace15/1
  state_d7_8/1 -> Bus Selector15/1, Bus Selector14/1
  Bus Selector13/1 -> To Workspace13/1
  Bus Selector14/1 -> To Workspace14/1
  Clock/1 -> To Workspace16/1
  Bus Selector18/1 -> To Workspace19/1
  Bus Selector19/1 -> To Workspace20/1
  Bus Selector20/1 -> To Workspace21/1
  u5_6/1 -> Bus Selector21/1, Bus Selector20/1
  Bus Selector21/1 -> To Workspace22/1
  Bus Selector23/1 -> To Workspace24/1
  u7_8/1 -> Bus Selector23/1, Bus Selector22/1
  u1_2/1 -> Bus Selector17/1, Bus Selector16/1
  Bus Selector17/1 -> To Workspace18/1
  Bus Selector16/1 -> To Workspace17/1
  u3_4/1 -> Bus Selector19/1, Bus Selector18/1
  Bus Selector22/1 -> To Workspace23/1

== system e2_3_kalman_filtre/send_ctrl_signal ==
  state1_2 : Inport
  state3_4 : Inport  Port=2
  state5_6 : Inport  Port=3
  state7_8 : Inport  Port=4
  control1_2 : Inport  Port=5
  control3_4 : Inport  Port=6
  control5_6 : Inport  Port=7
  control7_8 : Inport  Port=8
  Send Command 1 : Subsystem
  Send Command 2 : Subsystem
  Send Command 3 : Subsystem
  Send Command 4 : Subsystem
  Send Command 5 : Subsystem
  Send Command 6 : Subsystem
  Send Command 7 : Subsystem
  Send Command 8 : Subsystem
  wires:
  control1_2/1 -> Send Command 2/2(u), Send Command 1/2(u)
  state1_2/1 -> Send Command 2/1(pos), Send Command 1/1(pos)
  state3_4/1 -> Send Command 4/1(pos), Send Command 3/1(pos)
  control3_4/1 -> Send Command 4/2(u), Send Command 3/2(u)
  state5_6/1 -> Send Command 6/1(pos), Send Command 5/1(pos)
  control5_6/1 -> Send Command 6/2(u), Send Command 5/2(u)
  control7_8/1 -> Send Command 8/2(u), Send Command 7/2(u)
  state7_8/1 -> Send Command 8/1(pos), Send Command 7/1(pos)

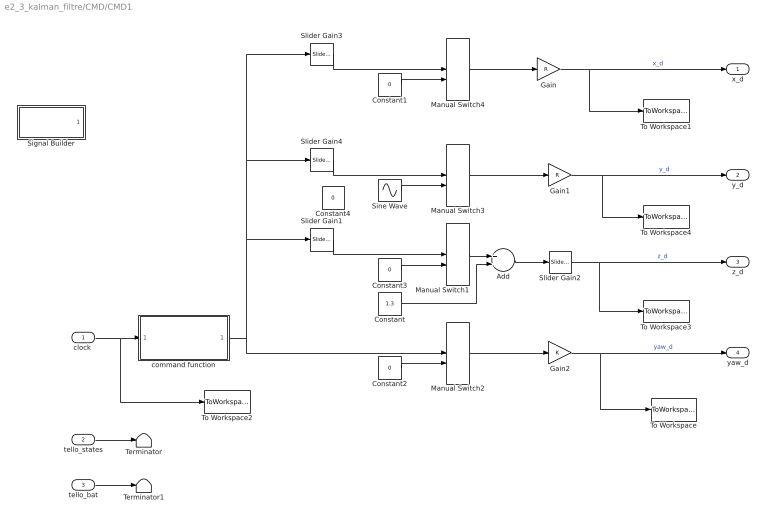
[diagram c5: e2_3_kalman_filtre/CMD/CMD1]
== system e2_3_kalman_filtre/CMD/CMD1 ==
  "clock " : Inport
  tello_states : Inport  Port=2
  tello_bat : Inport  Port=3
  Add : Sum
  Constant : Constant  Value=1.3
  Constant{1..4} (4 alike) : Constant  Value=0
  Gain : Gain  Gain=R
  Gain1 : Gain  Gain=R
  Gain2 : Gain
  Manual Switch{1..4} (4 alike) : ManualSwitch  CurrentSetting=0
  Signal Builder : Subsystem  Tag=STV Subsys  LoadFcn=sigbuilder_block('load');  StartFcn=sigbuilder_block('start');  StopFcn=sigbuilder_block('stop');  ClipboardFcn=sigbuilder_block('clipboard');  mask(Sigbuilder block){tuvar=[0:10]}
      mask help: Simulink:masks:SigbuilderBlock_MD
      mask init:
      | if ~strcmp(get_param(bdroot(gcbh),'SimulationStatus'),'stopped') tuvar = sigbuilder_block('maskInit'); end
  Sine Wave : Sin  Frequency=0.5  SampleTime=0
  Slider Gain1 : simulink/Math Operations/Slider Gain  gain=0.7  low=-2  high=2
  Slider Gain2 : simulink/Math Operations/Slider Gain  gain=-1  low=-2  high=2
  Slider Gain3 : simulink/Math Operations/Slider Gain  gain=0.5  low=-2  high=2
  Slider Gain4 : simulink/Math Operations/Slider Gain  gain=0.5  low=-2  high=2
  Terminator : Terminator
  Terminator1 : Terminator
  To Workspace : ToWorkspace  VariableName=yawd  SampleTime=-1
  To Workspace1 : ToWorkspace  VariableName=posxd  SampleTime=-1
  To Workspace2 : ToWorkspace  VariableName=time  SampleTime=-1
  To Workspace3 : ToWorkspace  VariableName=poszd  SampleTime=-1
  To Workspace4 : ToWorkspace  VariableName=posyd  SampleTime=-1
  command function : Subsystem
  x_d : Outport
  y_d : Outport  Port=2
  z_d : Outport  Port=3
  yaw_d : Outport  Port=4
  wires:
  Manual Switch1/1 -> Add/1
  Constant1/1 -> Manual Switch4/2
  Gain/1 -> x_d/1, To Workspace1/1  "x_d"
  Gain2/1 -> yaw_d/1, To Workspace/1  "yaw_d"
  Constant3/1 -> Manual Switch1/2
  Sine Wave/1 -> Manual Switch3/2
  Constant/1 -> Add/2
  command function/1(fcnCmd) -> Manual Switch2/1, Slider Gain4/1, Slider Gain3/1, Slider Gain1/1
  Manual Switch2/1 -> Gain2/1
  Slider Gain2/1 -> z_d/1, To Workspace3/1  "z_d"
  Manual Switch4/1 -> Gain/1
  "clock "/1 -> To Workspace2/1, command function/1(time)
  Constant2/1 -> Manual Switch2/2
  Manual Switch3/1 -> Gain1/1
  Add/1 -> Slider Gain2/1
  Gain1/1 -> y_d/1, To Workspace4/1  "y_d"
  tello_states/1 -> Terminator/1
  tello_bat/1 -> Terminator1/1
  Slider Gain1/1 -> Manual Switch1/1
  Slider Gain3/1 -> Manual Switch4/1
  Slider Gain4/1 -> Manual Switch3/1

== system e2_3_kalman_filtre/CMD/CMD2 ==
  "clock " : Inport
  tello_states : Inport  Port=2
  tello_bat : Inport  Port=3
  Bus Selector : BusSelector  OutputSignals=tello2_states.x2,tello2_states.y2,tello2_states.z2
  Constant : Constant  Value=sim_end_time
  Constant1 : Constant  Value=battery_threshold
  Constant2 : Constant  Value=z_d_for_land
  Constant3 : Constant  Value=0
  Constant4 : Constant  Value=UAV_NUM
  MATLAB Function : MATLAB Function  TreatAsAtomicUnit=on
  Manual Switch2 : ManualSwitch
  Sine Wave2 : Sin  Amplitude=0.3  Frequency=1.0
  Slider Gain3 : simulink/Math Operations/Slider Gain  gain=1  low=0  high=2
  Subsystem : Subsystem
  x_d : Outport
  y_d : Outport  Port=2
  z_d : Outport  Port=3
  yaw_d : Outport  Port=4
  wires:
  Manual Switch2/1 -> Slider Gain3/1
  Slider Gain3/1 -> yaw_d/1
  Sine Wave2/1 -> Manual Switch2/2
  Constant3/1 -> Manual Switch2/1
  "clock "/1 -> Subsystem/1(clock), MATLAB Function/4(timestamp)
  MATLAB Function/1(x_d_) -> x_d/1
  MATLAB Function/2(y_d_) -> y_d/1
  MATLAB Function/3(z_d_) -> z_d/1
  Subsystem/1("x ") -> MATLAB Function/1(x_d)
  Subsystem/2(y) -> MATLAB Function/2(y_d)
  Subsystem/3(z) -> MATLAB Function/3(z_d)
  tello_states/1 -> Bus Selector/1
  Bus Selector/1 -> MATLAB Function/5(x)  "<x2>"
  Bus Selector/2 -> MATLAB Function/6(y)  "<y2>"
  Bus Selector/3 -> MATLAB Function/7(z)  "<z2>"
  Constant/1 -> MATLAB Function/9(sim_time_end)
  Constant1/1 -> MATLAB Function/10(battery_threshold)
  Constant2/1 -> MATLAB Function/11(z_d_for_land)
  tello_bat/1 -> MATLAB Function/8(battery_status)
  Constant4/1 -> MATLAB Function/12(UAV_NUM)

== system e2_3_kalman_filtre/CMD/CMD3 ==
  "clock " : Inport
  tello_states : Inport  Port=2
  tello_bat : Inport  Port=3
  Bus Selector : BusSelector  OutputSignals=tello3_states.x3,tello3_states.y3,tello3_states.z3
  Constant : Constant  Value=sim_end_time
  Constant1 : Constant  Value=battery_threshold
  Constant2 : Constant  Value=z_d_for_land
  Constant3 : Constant  Value=0
  Constant4 : Constant  Value=UAV_NUM
  MATLAB Function : MATLAB Function  TreatAsAtomicUnit=on
  Manual Switch2 : ManualSwitch
  Sine Wave2 : Sin  Amplitude=0.3  Frequency=1.0
  Slider Gain3 : simulink/Math Operations/Slider Gain  gain=1  low=0  high=2
  Subsystem1 : Subsystem
  x_d : Outport
  y_d : Outport  Port=2
  z_d : Outport  Port=3
  yaw_d : Outport  Port=4
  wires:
  Manual Switch2/1 -> Slider Gain3/1
  Slider Gain3/1 -> yaw_d/1
  Sine Wave2/1 -> Manual Switch2/2
  Constant3/1 -> Manual Switch2/1
  Bus Selector/1 -> MATLAB Function/5(x)  "<x3>"
  MATLAB Function/2(y_d_) -> y_d/1
  Constant2/1 -> MATLAB Function/11(z_d_for_land)
  Subsystem1/3(z) -> MATLAB Function/3(z_d)
  Bus Selector/2 -> MATLAB Function/6(y)  "<y3>"
  Constant1/1 -> MATLAB Function/10(battery_threshold)
  MATLAB Function/3(z_d_) -> z_d/1
  tello_states/1 -> Bus Selector/1
  MATLAB Function/1(x_d_) -> x_d/1
  Constant4/1 -> MATLAB Function/12(UAV_NUM)
  Bus Selector/3 -> MATLAB Function/7(z)  "<z3>"
  Constant/1 -> MATLAB Function/9(sim_time_end)
  Subsystem1/1("x ") -> MATLAB Function/1(x_d)
  Subsystem1/2(y) -> MATLAB Function/2(y_d)
  "clock "/1 -> Subsystem1/1(clock), MATLAB Function/4(timestamp)
  tello_bat/1 -> MATLAB Function/8(battery_status)

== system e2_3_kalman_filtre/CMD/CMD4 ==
  "clock " : Inport
  tello_states : Inport  Port=2
  tello_bat : Inport  Port=3
  Bus Selector : BusSelector  OutputSignals=tello4_states.x4,tello4_states.y4,tello4_states.z4
  Constant : Constant  Value=sim_end_time
  Constant1 : Constant  Value=battery_threshold
  Constant2 : Constant  Value=z_d_for_land
  Constant3 : Constant  Value=0
  Constant4 : Constant  Value=UAV_NUM
  MATLAB Function : MATLAB Function  TreatAsAtomicUnit=on
  Manual Switch2 : ManualSwitch
  Sine Wave2 : Sin  Amplitude=0.3  Frequency=1.0
  Slider Gain3 : simulink/Math Operations/Slider Gain  gain=1  low=0  high=2
  Subsystem : Subsystem
  x_d : Outport
  y_d : Outport  Port=2
  z_d : Outport  Port=3
  yaw_d : Outport  Port=4
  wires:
  Manual Switch2/1 -> Slider Gain3/1
  Slider Gain3/1 -> yaw_d/1
  Sine Wave2/1 -> Manual Switch2/2
  Constant3/1 -> Manual Switch2/1
  Bus Selector/1 -> MATLAB Function/5(x)  "<x4>"
  MATLAB Function/2(y_d_) -> y_d/1
  Constant2/1 -> MATLAB Function/11(z_d_for_land)
  Subsystem/3(z) -> MATLAB Function/3(z_d)
  Bus Selector/2 -> MATLAB Function/6(y)  "<y4>"
  Constant1/1 -> MATLAB Function/10(battery_threshold)
  MATLAB Function/3(z_d_) -> z_d/1
  tello_states/1 -> Bus Selector/1
  MATLAB Function/1(x_d_) -> x_d/1
  Constant4/1 -> MATLAB Function/12(UAV_NUM)
  Bus Selector/3 -> MATLAB Function/7(z)  "<z4>"
  Constant/1 -> MATLAB Function/9(sim_time_end)
  Subsystem/1("x ") -> MATLAB Function/1(x_d)
  Subsystem/2(y) -> MATLAB Function/2(y_d)
  "clock "/1 -> Subsystem/1(clock), MATLAB Function/4(timestamp)
  tello_bat/1 -> MATLAB Function/8(battery_status)

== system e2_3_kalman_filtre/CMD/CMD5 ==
  "clock " : Inport
  Constant3 : Constant  Value=0
  Manual Switch2 : ManualSwitch
  Sine Wave2 : Sin  Amplitude=0.3  Frequency=1.0
  Slider Gain3 : simulink/Math Operations/Slider Gain  gain=1  low=0  high=2
  Subsystem : Subsystem
  x_d : Outport
  y_d : Outport  Port=2
  z_d : Outport  Port=3
  yaw_d : Outport  Port=4
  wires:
  Subsystem/1("x ") -> x_d/1
  Manual Switch2/1 -> Slider Gain3/1
  Slider Gain3/1 -> yaw_d/1
  Sine Wave2/1 -> Manual Switch2/2
  Constant3/1 -> Manual Switch2/1
  Subsystem/3(z) -> z_d/1
  "clock "/1 -> Subsystem/1(clock)
  Subsystem/2(y) -> y_d/1

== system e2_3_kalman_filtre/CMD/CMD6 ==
  "clock " : Inport
  Constant3 : Constant  Value=0
  Manual Switch2 : ManualSwitch
  Sine Wave2 : Sin  Amplitude=0.3  Frequency=1.0
  Slider Gain3 : simulink/Math Operations/Slider Gain  gain=1  low=0  high=2
  Subsystem : Subsystem
  x_d : Outport
  y_d : Outport  Port=2
  z_d : Outport  Port=3
  yaw_d : Outport  Port=4
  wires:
  Subsystem/1("x ") -> x_d/1
  Manual Switch2/1 -> Slider Gain3/1
  Slider Gain3/1 -> yaw_d/1
  Sine Wave2/1 -> Manual Switch2/2
  Constant3/1 -> Manual Switch2/1
  Subsystem/3(z) -> z_d/1
  "clock "/1 -> Subsystem/1(clock)
  Subsystem/2(y) -> y_d/1

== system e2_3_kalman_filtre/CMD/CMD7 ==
  "clock " : Inport
  Constant3 : Constant  Value=0
  Manual Switch2 : ManualSwitch
  Sine Wave2 : Sin  Amplitude=0.3  Frequency=1.0
  Slider Gain3 : simulink/Math Operations/Slider Gain  gain=1  low=0  high=2
  Subsystem : Subsystem
  x_d : Outport
  y_d : Outport  Port=2
  z_d : Outport  Port=3
  yaw_d : Outport  Port=4
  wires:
  Subsystem/1("x ") -> x_d/1
  Manual Switch2/1 -> Slider Gain3/1
  Slider Gain3/1 -> yaw_d/1
  Sine Wave2/1 -> Manual Switch2/2
  Constant3/1 -> Manual Switch2/1
  Subsystem/3(z) -> z_d/1
  "clock "/1 -> Subsystem/1(clock)
  Subsystem/2(y) -> y_d/1
